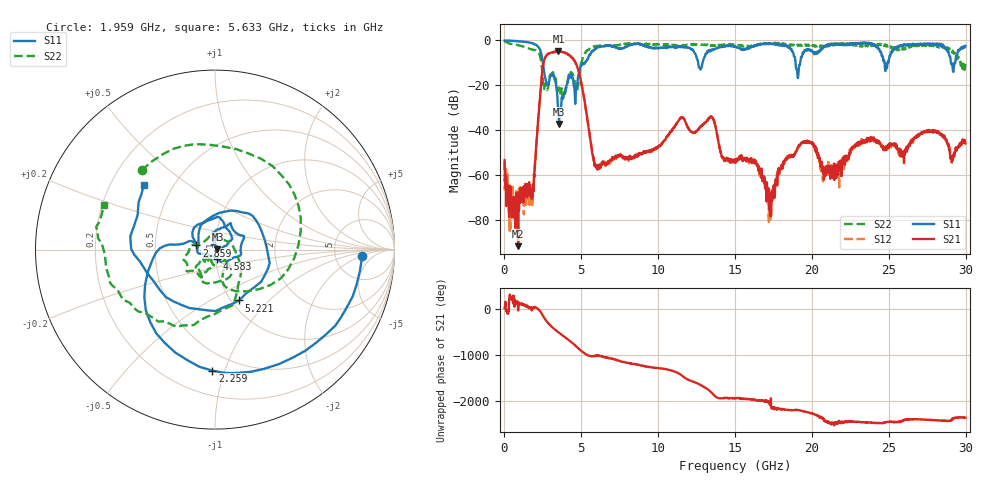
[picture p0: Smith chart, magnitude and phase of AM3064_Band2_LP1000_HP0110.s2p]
# Hz S DB R 50.0
!freq dBS11 angS11 dBS21 angS21 dBS12 angS12 dBS22 angS22
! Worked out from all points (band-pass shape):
!   1600 points, 10 MHz to 29.98 GHz, reference 50 ohm
!   highest |S21| = -4.83 dB at 3.515 GHz (marker M1); lowest = -91.6 dB at 891 MHz (marker M2)
!   |S21| within 3 dB of the highest: 2.639 GHz to 4.42 GHz (1.781 GHz wide, 50.5 % of centre)
!   lowest |S11| = -37.2 dB at 3.553 GHz (marker M3), VSWR 1.03, Z = 51.4 + j0.282 ohm
!   |S11| at or under -10 dB: 2.495 GHz to 5.234 GHz (2.738 GHz wide, 70.9 % of centre); 12.6 GHz to 12.88 GHz (284.1 MHz wide, 2.23 % of centre); 18.93 GHz to 19.23 GHz (300.9 MHz wide, 1.58 % of centre)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
!   |S22| runs from -24.9 to -0.2 dB; largest |S21 - S12| = 0.019
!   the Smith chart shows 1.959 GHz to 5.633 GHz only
!   S11 on the Smith chart (normalised r, x): 1.959 GHz: 9.68, -2.17; 2.259 GHz: 0.37, -0.91; 2.859 GHz: 0.81, +0.04; 4.583 GHz: 1.02, -0.11; 5.221 GHz: 1.09, -0.68; 5.633 GHz: 0.34, +0.35
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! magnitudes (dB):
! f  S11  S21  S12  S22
! 10 MHz  0.0  -53.2  -53.8  -0.2
! 891 MHz  -0.4  -91.6  -74.9  -2.2
! 1.959 GHz  -1.7  -57.3  -58.5  -4.4
! 2.259 GHz  -3.4  -29.3  -29.3  -5.9
! 2.859 GHz  -19.5  -5.9  -5.9  -19.9
! 3.515 GHz  -32.1  -4.8  -5.0  -22.4
! 3.553 GHz  -37.2  -5.1  -4.9  -21.2
! 4.583 GHz  -25.1  -9.4  -9.3  -20.3
! 5.015 GHz  -11.0  -19.4  -19.4  -9.6
! 5.221 GHz  -10.1  -27.3  -27.3  -5.8
! 5.633 GHz  -5.4  -46.3  -46.3  -3.5
! 6.083 GHz  -3.1  -55.6  -56.6  -2.5
! 10 GHz  -3.4  -47.3  -47.3  -1.8
! 13.43 GHz  -4.5  -33.9  -33.9  -2.5
! 15 GHz  -2.5  -54.3  -53.9  -1.8
! 16.34 GHz  -2.4  -54.7  -53.6  -2.4
! 17.27 GHz  -1.4  -71.4  -68.2  -1.3
! 19.09 GHz  -16.8  -47.7  -47.9  -2.3
! 19.99 GHz  -4.5  -45.9  -46.0  -1.9
! 20.78 GHz  -2.8  -61.9  -55.5  -2.9
! 25 GHz  -9.0  -48.0  -47.4  -2.3
! 29.98 GHz  -2.5  -45.9  -45.4  -10.5
